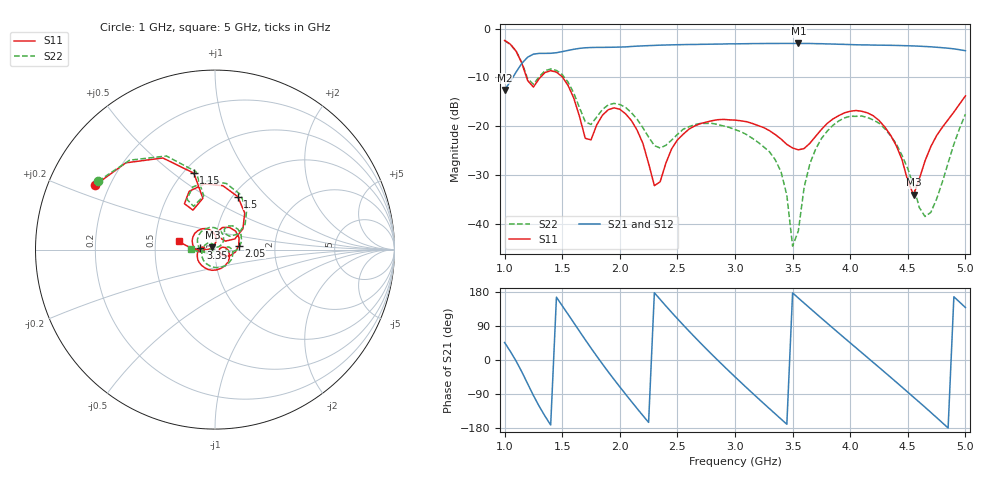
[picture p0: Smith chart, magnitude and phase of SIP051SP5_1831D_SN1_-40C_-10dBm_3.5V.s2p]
# GHz  S  dB  R  50
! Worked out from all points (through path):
!   81 points, 1 GHz to 5 GHz, reference 50 ohm
!   highest |S21| = -3.02 dB at 3.55 GHz (marker M1); lowest = -12.6 dB at 1 GHz (marker M2)
!   lowest |S11| = -34.1 dB at 4.55 GHz (marker M3), VSWR 1.04, Z = 48.5 + j1.29 ohm
!   |S11| at or under -10 dB: 1.191 GHz to 1.31 GHz (119.1 MHz wide, 9.53 % of centre); 1.504 GHz to end of sweep
!   |S22| runs from -44.6 to -2.4 dB; largest |S21 - S12| = 0.0021
!   S11 on the Smith chart (normalised r, x): 1 GHz: 0.15, +0.25; 1.15 GHz: 0.56, +0.60; 1.5 GHz: 1.06, +0.69; 2.05 GHz: 1.30, +0.06; 3.35 GHz: 0.85, +0.02; 5 GHz: 0.67, +0.06
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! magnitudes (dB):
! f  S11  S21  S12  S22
! 1 GHz  -2.4  -12.6  -12.6  -2.4
! 1.15 GHz  -7.1  -7.1  -7.1  -7.0
! 1.25 GHz  -12.0  -5.2  -5.2  -11.4
! 1.5 GHz  -9.9  -4.7  -4.7  -9.4
! 1.7 GHz  -22.5  -3.9  -3.9  -19.1
! 1.9 GHz  -16.6  -3.8  -3.8  -15.6
! 2.05 GHz  -17.5  -3.7  -3.7  -16.1
! 2.3 GHz  -32.2  -3.4  -3.4  -24.0
! 2.35 GHz  -31.4  -3.4  -3.4  -24.5
! 2.6 GHz  -20.6  -3.2  -3.2  -20.1
! 3 GHz  -18.8  -3.1  -3.1  -20.7
! 3.35 GHz  -21.7  -3.0  -3.0  -26.9
! 3.45 GHz  -23.7  -3.0  -3.0  -34.2
! 3.5 GHz  -24.5  -3.0  -3.0  -44.6
! 3.55 GHz  -24.9  -3.0  -3.0  -41.5
! 3.6 GHz  -24.6  -3.0  -3.0  -32.6
! 3.7 GHz  -22.1  -3.1  -3.1  -24.7
! 4 GHz  -16.9  -3.3  -3.3  -18.0
! 4.35 GHz  -21.8  -3.4  -3.4  -21.9
! 4.55 GHz  -34.1  -3.5  -3.5  -32.3
! 4.7 GHz  -24.2  -3.7  -3.7  -37.7
! 5 GHz  -13.8  -4.5  -4.5  -17.5
